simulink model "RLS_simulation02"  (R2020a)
settings: Solver=ode45  StartTime=0.0  StopTime=2000  RelTol=1e-3  EnableMultiTasking=on
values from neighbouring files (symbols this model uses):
  Ts = 0.2    [init_model.m]
libraries: ctrlSharedLib x1

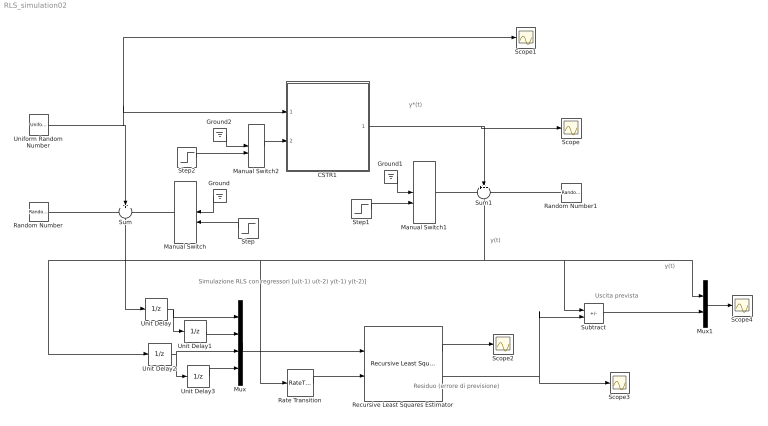
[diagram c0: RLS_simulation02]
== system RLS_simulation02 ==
  note: Residuo (errore di previsione)
  note: y(t)
  note: y*(t)
  note: Uscita prevista
  note: Simulazione RLS con regressori [u(t-1) u(t-2) y(t-1) y(t-2)]
  note: y(t)
  CSTR1 : Subsystem
  Ground : Ground
  Ground1 : Ground
  Ground2 : Ground
  Manual Switch : ManualSwitch
  Manual Switch1 : ManualSwitch  CurrentSetting=0
  Manual Switch2 : ManualSwitch
  Mux : Mux
  Mux1 : Mux  Inputs=2
  Random Number : RandomNumber  Variance=0.0001  Seed=1  SampleTime=Ts
  Random Number1 : RandomNumber  Variance=0.0005  Seed=2  SampleTime=Ts
  Rate Transition : RateTransition
  Recursive Least Squares Estimator : ctrlSharedLib/Recursive Least Squares Estimator  InitialEstimateSource=None  InitialParameterData=4  P0=1e4  InitialRegressors=0  InitialOutputs=0  History=Infinite  WindowLength=200  EstimationMethod=Forgetting Factor  AdaptationParameter=1  HasTimeVaryingAdaptationParameter=off  NormalizationBias=eps  OutputError=on  OutputP=off  AddEnablePort=off  InputProcessing=Sample-based  Ts=Ts
  Scope{,1..4} (5 alike) : Scope
  Step : Step  Time=900  SampleTime=0
  Step1 : Step  Time=1000  After=10  SampleTime=0
  Step2 : Step  Time=1000  SampleTime=0
  Subtract : Sum  Inputs=+-
  Sum : Sum  Inputs=+++  SaturateOnIntegerOverflow=on
  Sum1 : Sum  Inputs=+++  SaturateOnIntegerOverflow=on
  Uniform Random Number : UniformRandomNumber  Minimum=0  Maximum=4  SampleTime=20
  Unit Delay{,1..3} (4 alike) : UnitDelay  SampleTime=Ts  HasFrameUpgradeWarning=on
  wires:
  Uniform Random Number/1 -> CSTR1/1(w), Scope1/1, Sum/2
  Random Number/1 -> Sum/1
  Manual Switch/1 -> Sum/3
  Sum/1 -> Unit Delay/1
  Ground/1 -> Manual Switch/1
  Step/1 -> Manual Switch/2
  Ground1/1 -> Manual Switch1/1
  Step1/1 -> Manual Switch1/2
  CSTR1/1(Cb) -> Scope/1, Sum1/2
  Manual Switch1/1 -> Sum1/1
  Random Number1/1 -> Sum1/3
  Unit Delay/1 -> Unit Delay1/1, Mux/1
  Unit Delay1/1 -> Mux/2
  Unit Delay2/1 -> Mux/3, Unit Delay3/1
  Unit Delay3/1 -> Mux/4
  Mux/1 -> Recursive Least Squares Estimator/1
  Rate Transition/1 -> Recursive Least Squares Estimator/2
  Recursive Least Squares Estimator/1 -> Scope2/1
  Recursive Least Squares Estimator/2 -> Subtract/2, Scope3/1
  Sum1/1 -> Subtract/1, Mux1/1, Rate Transition/1, Unit Delay2/1
  Subtract/1 -> Mux1/2
  Mux1/1 -> Scope4/1
  Step2/1 -> Manual Switch2/2
  Manual Switch2/1 -> CSTR1/2(f)
  Ground2/1 -> Manual Switch2/1

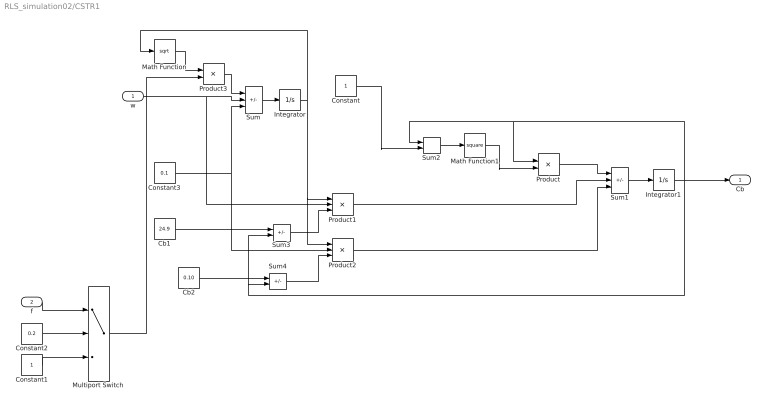
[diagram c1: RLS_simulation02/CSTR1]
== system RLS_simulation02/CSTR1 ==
  w : Inport
  f : Inport  Port=2
  Cb1 : Constant  Value=24.9
  Cb2 : Constant  Value=0.10
  Constant : Constant
  Constant1 : Constant
  Constant2 : Constant  Value=0.2
  Constant3 : Constant  Value=0.1
  Integrator : Integrator  InitialCondition=30  LimitOutput=on  LowerSaturationLimit=1
  Integrator1 : Integrator  InitialCondition=22
  Math Function : Math  Operator=sqrt
  Math Function1 : Math  Operator=square
  Multiport Switch : MultiPortSwitch  DataPortOrder=Zero-based contiguous  Inputs=2  zeroidx=on
  Product : Product  Inputs=*/  SaturateOnIntegerOverflow=on
  Product1 : Product  Inputs=/**  SaturateOnIntegerOverflow=on
  Product2 : Product  Inputs=/**  SaturateOnIntegerOverflow=on
  Product3 : Product
  Sum : Sum  Inputs=-++  SaturateOnIntegerOverflow=on
  Sum1 : Sum  Inputs=-++  SaturateOnIntegerOverflow=on
  Sum2 : Sum  SaturateOnIntegerOverflow=on
  Sum3 : Sum  Inputs=+-  SaturateOnIntegerOverflow=on
  Sum4 : Sum  Inputs=+-  SaturateOnIntegerOverflow=on
  Cb : Outport
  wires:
  Sum/1 -> Integrator/1
  Product3/1 -> Sum/1
  Math Function/1 -> Product3/1
  Integrator/1 -> Math Function/1, Product1/1, Product2/1
  Sum3/1 -> Product1/3
  Sum4/1 -> Product2/3
  Sum2/1 -> Math Function1/1
  Sum1/1 -> Integrator1/1
  Math Function1/1 -> Product/2
  Product/1 -> Sum1/1
  Product1/1 -> Sum1/2
  Product2/1 -> Sum1/3
  w/1 -> Sum/2, Product1/2
  Constant3/1 -> Product2/2, Sum/3
  Integrator1/1 -> Sum3/2, Sum4/2, Sum2/1, Product/1, Cb/1
  Constant1/1 -> Multiport Switch/3
  f/1 -> Multiport Switch/1
  Constant2/1 -> Multiport Switch/2
  Cb2/1 -> Sum4/1
  Cb1/1 -> Sum3/1
  Constant/1 -> Sum2/2
  Multiport Switch/1 -> Product3/2
